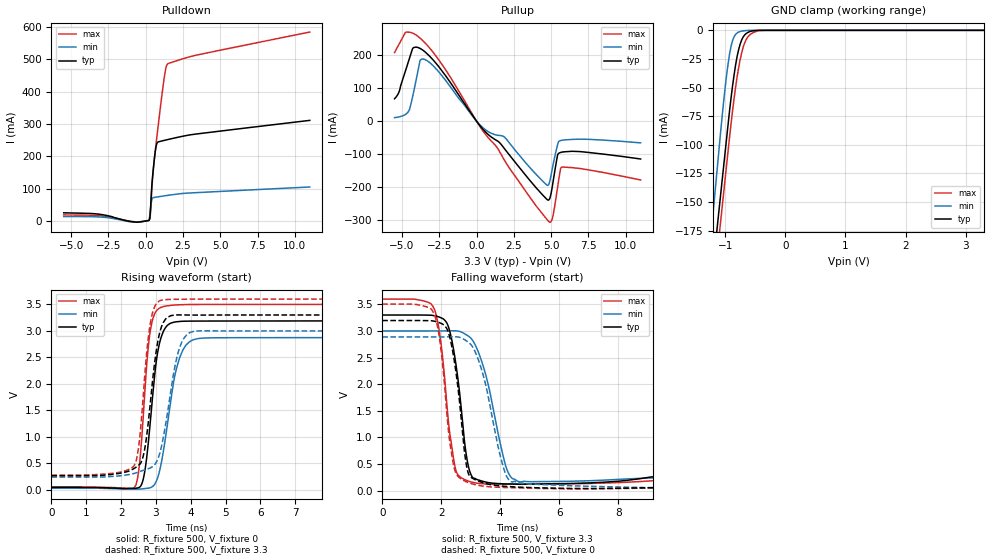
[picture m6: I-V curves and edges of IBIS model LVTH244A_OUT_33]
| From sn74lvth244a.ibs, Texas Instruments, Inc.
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[Model]   LVTH244A_OUT_33
Model_type  3-state
Enable   Active-Low
Vref =   0
Rref =   500
Cref =   50p
Vmeas =   1.5
| variable   typ   min   max
C_comp   5.67pF   4.63pF   7.98pF
| C_pullup   4.98pF   0.16pF   7.32pF
| C_pulldown   9.47pF   2.03pF   32.17pF
| C_tri-state   5.67pF   4.63pF   7.98pF
[Temperature Range]   40   -40   100
| Ambient temperature   25   -40   85
[Voltage range]   3.3   3   3.6
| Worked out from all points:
|   slope of the pulldown table from 0 to 0.495 V, typ, clamps not added: 3.18 ohm
|   slope of the pullup table from 0 to 0.495 V, typ, clamps not added: 17.9 ohm
|   GND clamp passes 1 mA (typ) near -0.58 V on its own axis
|   rising waveform, R_fixture 500, V_fixture 0: 20-80 % time 295ps typ, 418ps min, 235ps max; typ from 0.041 V to 3.19 V
|   falling waveform, R_fixture 500, V_fixture 3.3: 20-80 % time 396ps typ, 681ps min, 376ps max; typ from 3.3 V to 0.26 V
|   rising waveform, R_fixture 500, V_fixture 3.3: 20-80 % time 323ps typ, 434ps min, 265ps max; typ from 0.261 V to 3.3 V
|   falling waveform, R_fixture 500, V_fixture 0: 20-80 % time 396ps typ, 682ps min, 384ps max; typ from 3.2 V to 0.041 V
[GND Clamp]
| LVTH244A_OUT_33
|   Voltage   I(typ)   I(min)   I(max)
-5.5V     -2.861A    -3.034A    -2.892A
-1.24V    -226.4mA   -182.9mA   -251mA
-1.21V    -211.3mA   -165.7mA   -235.5mA
-1.17V    -191.4mA   -142.9mA   -215.1mA
-1.075V   -144mA     -89.19mA   -167.4mA
-975mV    -94.37mA   -39.09mA   -117.7mA
-925mV    -69.94mA   -20.46mA   -92.96mA
-875mV    -48.14mA   -8.719mA   -69.85mA
-800mV    -22.75mA   -2.299mA   -40.47mA
-725mV    -8.466mA   -746.4uA   -19.69mA
-575mV    -873.9uA   -11.47uA   -3.26mA
3.3V      32.83pA    25.31pA    1.688nA
[Pulldown]
| LVTH244A_OUT_33
|   Voltage   I(typ)   I(min)   I(max)
-5.5V     24.91mA    13.36mA    18.33mA
-3.15V    20.78mA    12.26mA    15.98mA
-695mV    -3.712mA   -4.073mA   -3.095mA
245mV     3.449mA    7.854mA    3.6mA
315mV     33.12mA    35.71mA    21.95mA
425mV     118.9mA    67.74mA    109.9mA
580mV     192.7mA    72.62mA    190.9mA
710mV     233.6mA    73.58mA    245.4mA
1.245V    249.3mA    77.41mA    444.8mA
1.365V    250.6mA    78.23mA    476mA
1.475V    251.8mA    78.98mA    486.2mA
11V       311.3mA    104.9mA    584.7mA
[Pullup]
| LVTH244A_OUT_33
|   Voltage   I(typ)   I(min)   I(max)
-5.5V     67.92mA    10.82mA    207.4mA
-4.615V   173.6mA    26.44mA    269.3mA
-4.28V    220.1mA    75.69mA    266.1mA
-3.79V    220mA      182.9mA    251.2mA
-3.465V   209.8mA    186.5mA    237.2mA
270mV     -15.96mA   -13.16mA   -19.22mA
1.855V    -82.19mA   -47.41mA   -116.7mA
4.89V     -235.3mA   -184.7mA   -304.8mA
5.11V     -188.9mA   -136.1mA   -288.5mA
5.435V    -102.2mA   -70.96mA   -199.1mA
5.69V     -93.81mA   -57.8mA    -139.6mA
11V       -114.3mA   -65.47mA   -177.8mA
[Ramp]
| LVTH244A_OUT_33
| variable   typ   min   max
dV/dt_r   1.90/3.05E-10   1.72/4.25E-10   2.09/2.40E-10
dV/dt_f   1.91/4.19E-10   1.70/7.03E-10   2.09/4.02E-10
R_load = 500
[Rising Waveform]
| LVTH244A_OUT_33
R_fixture =   500
C_fixture =   0
L_fixture =   0
V_fixture =   0
V_fixture_min = 0
V_fixture_max = 0
|   Time   V(typ)   V(min)   V(max)
0s        41.42mV    26.97mV    51.02mV
2.405ns   23.89mV    7.907mV    61.38mV
2.525ns   43.77mV    9.77mV     461.6mV
2.65ns    236.7mV    16.2mV     1.518V
2.87ns    1.504V     44.28mV    3.112V
3.095ns   2.741V     325.8mV    3.426V
3.41ns    3.14V      1.601V     3.48V
3.775ns   3.181V     2.636V     3.494V
4.39ns    3.184V     2.864V     3.498V
50ns      3.188V     2.873V     3.5V
[Falling Waveform]
| LVTH244A_OUT_33
R_fixture =   500
C_fixture =   0
L_fixture =   0
V_fixture =   3.3
V_fixture_min = 3
V_fixture_max = 3.6
|   Time   V(typ)   V(min)   V(max)
0s        3.3V       3V         3.6V
1.71ns    3.293V     3.001V     3.47V
1.95ns    3.258V     3.001V     2.943V
2.19ns    3.152V     3.002V     1.633V
2.52ns    2.293V     3.001V     343.3mV
2.905ns   499.4mV    2.91V      182.2mV
3.29ns    195.2mV    2.56V      134.6mV
4.185ns   126mV      464.2mV    118.8mV
4.675ns   122.7mV    164.6mV    119.1mV
50ns      260.2mV    235.1mV    272.9mV
[Rising Waveform]
| LVTH244A_OUT_33
R_fixture =   500
C_fixture =   0
L_fixture =   0
V_fixture =   3.3
V_fixture_min = 3
V_fixture_max = 3.6
|   Time   V(typ)   V(min)   V(max)
0s        260.8mV    235.5mV    273.3mV
2.365ns   395.5mV    302.7mV    444.5mV
2.5ns     456.5mV    332.3mV    784.7mV
2.635ns   631.1mV    363.2mV    1.758V
2.845ns   1.671V     411.1mV    3.163V
3.04ns    2.744V     552.4mV    3.532V
3.24ns    3.186V     1.083V     3.589V
3.66ns    3.301V     2.64V      3.596V
4.15ns    3.298V     2.997V     3.599V
50ns      3.3V       3V         3.6V
[Falling Waveform]
| LVTH244A_OUT_33
R_fixture =   500
C_fixture =   0
L_fixture =   0
V_fixture =   0
V_fixture_min = 0
V_fixture_max = 0
|   Time   V(typ)   V(min)   V(max)
0s        3.196V     2.888V     3.505V
1.715ns   3.188V     2.888V     3.369V
1.955ns   3.153V     2.889V     2.812V
2.185ns   3.05V      2.889V     1.488V
2.46ns    2.38V      2.891V     384.7mV
2.89ns    382.8mV    2.801V     157.7mV
3.425ns   146.4mV    2.168V     84.14mV
4.175ns   79.47mV    321.3mV    57.91mV
4.705ns   63.71mV    137.9mV    49.89mV
50ns      41.43mV    26.96mV    51.09mV
